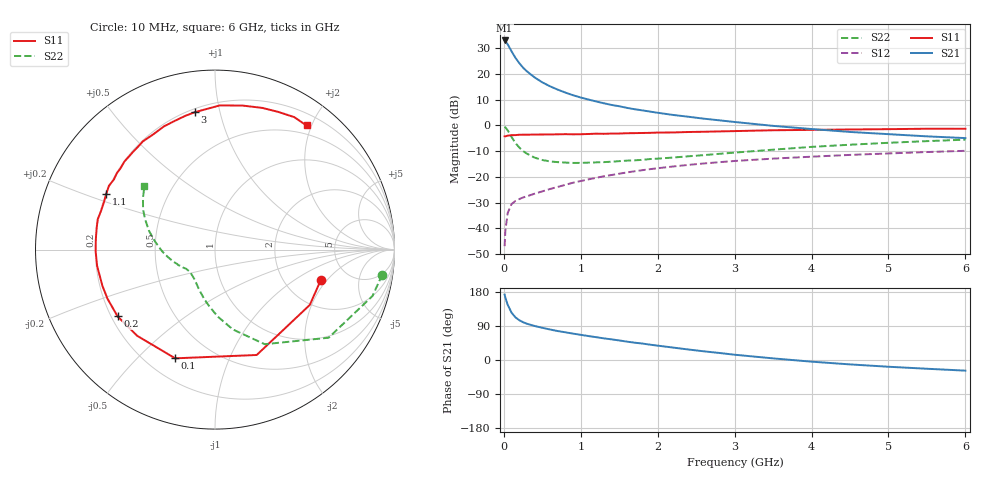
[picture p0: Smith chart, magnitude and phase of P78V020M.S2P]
! SIEMENS Small Signal Semiconductors
! BFP196
! Si NPN RF Bipolar Junction Transistor in SOT143
! VCE = 8 V  IC = 20 mA
! Common Emitter S-Parameters:  May  1996
# GHz  S  MA  R  50
!  f  S11  S21  S12  S22
! GHz  MAG  ANG  MAG  ANG  MAG  ANG  MAG  ANG
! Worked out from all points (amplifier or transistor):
!   36 points, 10 MHz to 6 GHz, reference 50 ohm
!   highest |S21| = 33.0 dB at 10 MHz (marker M1)
!   |S21| within 3 dB of that: start of sweep to 77.67 MHz
!   unconditionally stable (mu >= 1): 729 MHz to 4.087 GHz
!   at 250 MHz: K = 0.57, MSG = 25.2 dB, |S12| = -28.0 dB
!   at 1.4 GHz: K = 1.11, MAG = 11.6 dB, |S12| = -19.3 dB
!   at 6 GHz: K = 0.96, MSG = 2.5 dB, |S12| = -9.9 dB
!   S11 on the Smith chart (normalised r, x): 10 MHz: 3.18, -1.71; 100 MHz: 0.31, -0.65; 200 MHz: 0.23, -0.30; 1.1 GHz: 0.20, +0.23; 3 GHz: 0.22, +0.84; 6 GHz: 0.36, +1.92
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0.01  0.6137 -15.9  44.64 172.7  0.0045 83.9  0.9421 -8.5
0.02  0.6115 -30.3  42.9 164.4  0.0091 76.6  0.915 -16.4
0.05  0.6315 -68.4  37.55 145.8  0.0198 62.3  0.8011 -37.8
0.1  0.6451 -110.1  27.5 124.9  0.0296 48.5  0.5953 -62.3
0.15  0.6471 -132.1  20.59 112.7  0.034 41.7  0.4558 -77.4
0.2  0.658 -145.6  16.25 105.1  0.037 41.0  0.3725 -87.8
0.25  0.6585 -155.4  13.23 99.7  0.0397 40.2  0.316 -96.0
0.3  0.6591 -162.1  11.2 95.7  0.0419 41.9  0.2817 -102.4
0.4  0.6631 -172.1  8.548 89.8  0.0471 43.9  0.2365 -112.5
0.5  0.6651 -179.3  6.85 85.0  0.0522 46.3  0.2123 -119.9
0.6  0.6664 175.1  5.745 80.5  0.058 48.2  0.1994 -125.6
0.7  0.6703 169.7  4.95 76.4  0.0637 49.6  0.1932 -130.3
0.9  0.6705 161.3  3.848 69.6  0.077 51.0  0.1864 -137.3
1.1  0.6802 153.1  3.172 63.2  0.0893 51.7  0.189 -142.0
1.3  0.6855 145.3  2.689 57.1  0.1026 51.1  0.1932 -146.5
1.6  0.7037 135.9  2.187 48.5  0.1219 49.3  0.2065 -152.2
2.2  0.7285 118.2  1.594 32.8  0.159 43.4  0.2373 -162.7
3  0.7739 98.3  1.164 13.9  0.2034 33.9  0.2957 -178.4
3.5  0.804 88.0  0.978 4.3  0.226 27.8  0.3373 172.3
4.5  0.8323 71.5  0.745 -11.6  0.2669 16.7  0.421 157.1
5.5  0.86 59.1  0.612 -23.1  0.3032 6.1  0.4942 144.3
6  0.8591 53.6  0.566 -28.1  0.3205 0.3  0.5275 138.2
